FUNCTION "PERIPHERAL" : VOID
TITLE =INPUT/OUTPUT PERIPHERAL
AUTHOR : Esposito
FAMILY : EGAL_srl
NAME : PERIF_P
VERSION : 0.1

BEGIN
NETWORK
TITLE =SIGNALS PRESS FOR PERIPHERICAL
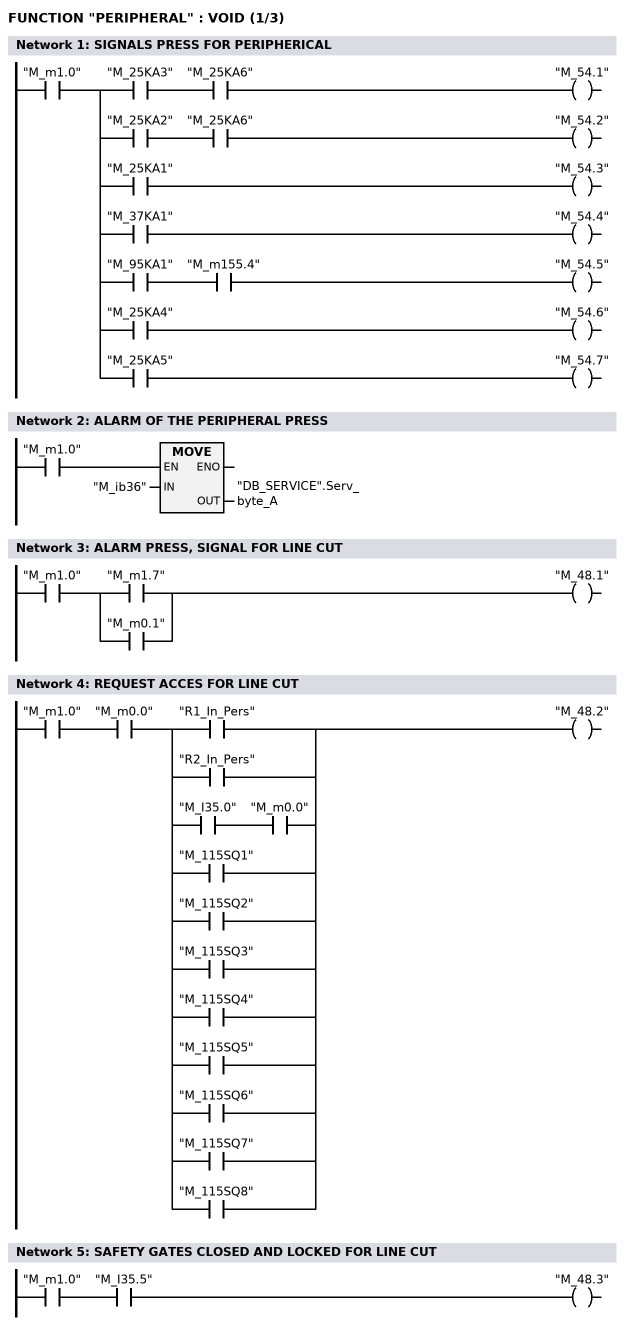
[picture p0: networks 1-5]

      U     "M_m1.0";
      =     L      0.0;
      U     L      0.0;
      U     "M_25KA3";
      U     "M_25KA6";
      =     "M_54.1";
      U     L      0.0;
      U     "M_25KA2";
      U     "M_25KA6";
      =     "M_54.2";
      U     L      0.0;
      U     "M_25KA1";
      =     "M_54.3";
      U     L      0.0;
      U     "M_37KA1";
      =     "M_54.4";
      U     L      0.0;
      U     "M_95KA1";
      U     "M_m155.4";
      =     "M_54.5";
      U     L      0.0;
      U     "M_25KA4";
      =     "M_54.6";
      U     L      0.0;
      U     "M_25KA5";
      =     "M_54.7";
NETWORK
TITLE =ALARM OF THE PERIPHERAL PRESS

      U     "M_m1.0";
      SPBNB _001;
      L     "M_ib36";
      T     "DB_SERVICE".Serv_byte_A;
_001: NOP   0;
NETWORK
TITLE =ALARM PRESS, SIGNAL FOR LINE CUT

      U     "M_m1.0";
      U(    ;
      O     "M_m1.7";
      O     "M_m0.1";
      )     ;
      =     "M_48.1";
NETWORK
TITLE =REQUEST ACCES FOR LINE CUT

      U     "M_m1.0";
      U     "M_m0.0";
      U(    ;
      O     "R1_In_Pers";
      O     "R2_In_Pers";
      O     ;
      U     "M_I35.0";
      U     "M_m0.0";
      O     "M_115SQ1";
      O     "M_115SQ2";
      O     "M_115SQ3";
      O     "M_115SQ4";
      O     "M_115SQ5";
      O     "M_115SQ6";
      O     "M_115SQ7";
      O     "M_115SQ8";
      )     ;
      =     "M_48.2";
NETWORK
TITLE =SAFETY GATES CLOSED AND LOCKED FOR LINE CUT

      U     "M_m1.0";
      U     "M_I35.5";
      =     "M_48.3";
NETWORK
TITLE =OPZIONI FUNZIONAMENTO  ROBOT- TAVOLA DI CENTRAGGIO
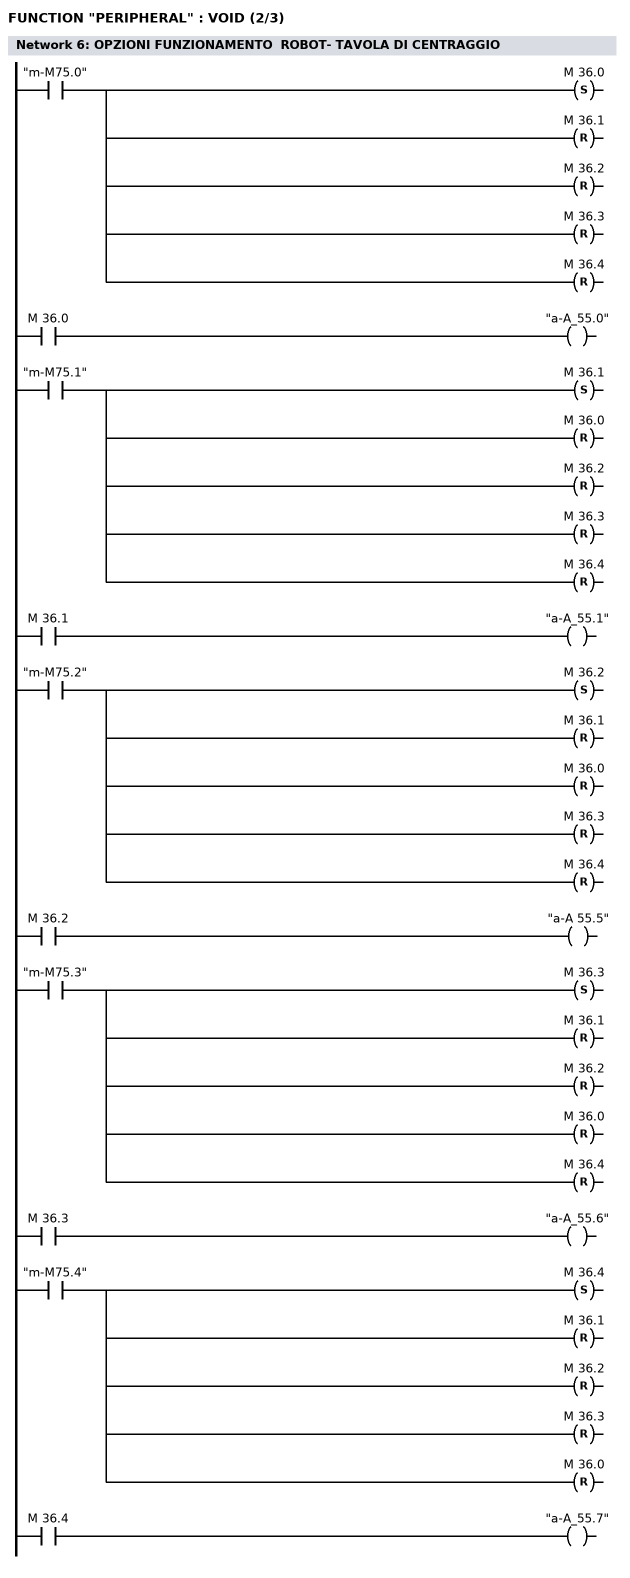
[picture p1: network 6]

// CICLO 1"ROBOT 1/ ROBOT 2
      U     "m-M75.0";
      S     M     36.0;
      R     M     36.1;
      R     M     36.2;
      R     M     36.3;
      R     M     36.4;

      U     M     36.0;
      =     "a-A_55.0";

// Ciclo 2 "paller 1/pallet 2"
      U     "m-M75.1";
      S     M     36.1;
      R     M     36.0;
      R     M     36.2;
      R     M     36.3;
      R     M     36.4;

      U     M     36.1;
      =     "a-A_55.1";

// Ciclo 3 "pallet 2/pallet 1"
      U     "m-M75.2";
      S     M     36.2;
      R     M     36.1;
      R     M     36.0;
      R     M     36.3;
      R     M     36.4;

      U     M     36.2;
      =     "a-A 55.5";

// Ciclo 4 "robot 1"
      U     "m-M75.3";
      S     M     36.3;
      R     M     36.1;
      R     M     36.2;
      R     M     36.0;
      R     M     36.4;

      U     M     36.3;
      =     "a-A_55.6";

// Ciclo 5 " robot 2"
      U     "m-M75.4";
      S     M     36.4;
      R     M     36.1;
      R     M     36.2;
      R     M     36.3;
      R     M     36.0;

      U     M     36.4;
      =     "a-A_55.7";

NETWORK
TITLE =SELEZIONE COMANDO FEEDER DA OP 37
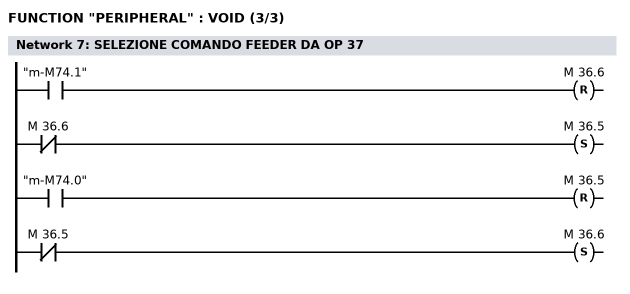
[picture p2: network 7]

// Comando da tavola
      U     "m-M74.1";
      R     M     36.6;
      UN    M     36.6;
      S     M     36.5;

// Comando da pressa
      U     "m-M74.0";
      R     M     36.5;
      UN    M     36.5;
      S     M     36.6;

END_FUNCTION

